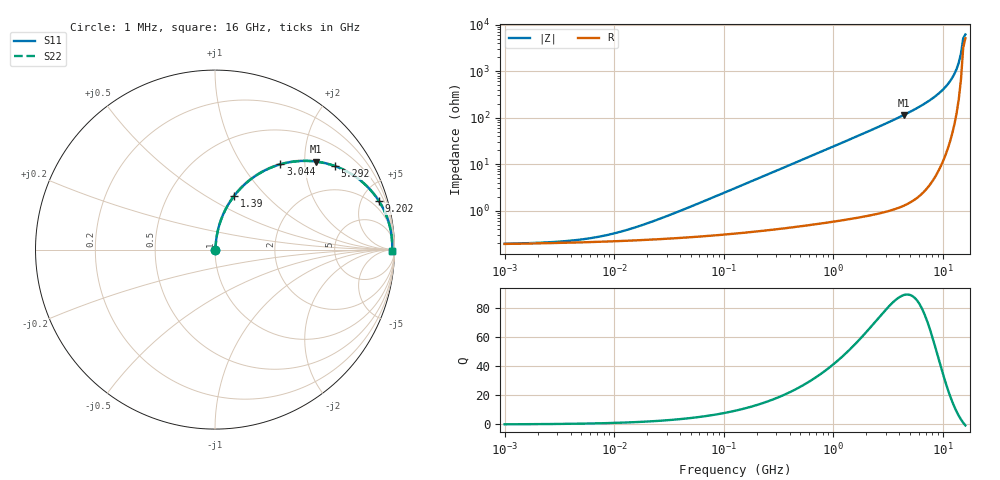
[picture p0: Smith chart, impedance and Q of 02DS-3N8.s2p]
# MHz S MA R 50
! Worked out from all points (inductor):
!   211 points, 1 MHz to 16 GHz, reference 50 ohm
!   read as one part in series: L = 3.8 nH near 31.73 MHz
!   highest Q = 89.1 at 4.401 GHz (marker M1), where L = 4.12 nH
!   self-resonance near 15.28 GHz
!   S11 on the Smith chart (normalised r, x): 1 MHz: 1.00, +0.00; 1.39 GHz: 1.01, +0.67; 3.044 GHz: 1.02, +1.51; 5.292 GHz: 1.03, +2.85; 9.202 GHz: 1.15, +6.68; 16 GHz: open
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1  0.001936 7.1  0.9981 -0.0  0.9981 -0.0  0.001936 7.1
2.63276  0.002095 17.4  0.998 -0.0  0.998 -0.0  0.002095 17.4
5.25662  0.00243 31.0  0.9979 -0.1  0.9979 -0.1  0.00243 31.0
11.5091  0.003527 50.9  0.9978 -0.2  0.9978 -0.2  0.003527 50.9
26.3872  0.00674 68.5  0.9975 -0.4  0.9975 -0.4  0.00674 68.5
132.458  0.03168 82.3  0.9963 -1.8  0.9963 -1.8  0.03168 82.3
333.021  0.07908 82.5  0.9928 -4.5  0.9928 -4.5  0.07908 82.5
664.915  0.1564 79.2  0.9828 -9.0  0.9828 -9.0  0.1564 79.2
1390.21  0.3155 70.5  0.9428 -18.4  0.9428 -18.4  0.3155 70.5
2105.02  0.4528 62.2  0.8847 -26.9  0.8847 -26.9  0.4528 62.2
3043.78  0.599 52.5  0.7932 -36.8  0.7932 -36.8  0.599 52.5
3187.38  0.618 51.1  0.7786 -38.2  0.7786 -38.2  0.618 51.1
4401.2  0.7477 41.0  0.6557 -48.4  0.6557 -48.4  0.7477 41.0
5292.36  0.8143 34.8  0.5713 -54.5  0.5713 -54.5  0.8143 34.8
7307.8  0.9073 24.1  0.4076 -65.1  0.4076 -65.1  0.9073 24.1
9202.05  0.9521 16.5  0.2849 -72.2  0.2849 -72.2  0.9521 16.5
11065.3  0.9748 10.7  0.1863 -76.9  0.1863 -76.9  0.9748 10.7
12706.4  0.9844 6.5  0.1129 -78.8  0.1129 -78.8  0.9844 6.5
13933.5  0.9873 3.7  0.06465 -76.8  0.06465 -76.8  0.9873 3.7
14590.9  0.9877 2.3  0.0411 -71.5  0.0411 -71.5  0.9877 2.3
15279.2  0.9875 0.9  0.01963 -49.9  0.01963 -49.9  0.9875 0.9
16000  0.9866 -0.5  0.01612 33.3  0.01612 33.3  0.9866 -0.5
